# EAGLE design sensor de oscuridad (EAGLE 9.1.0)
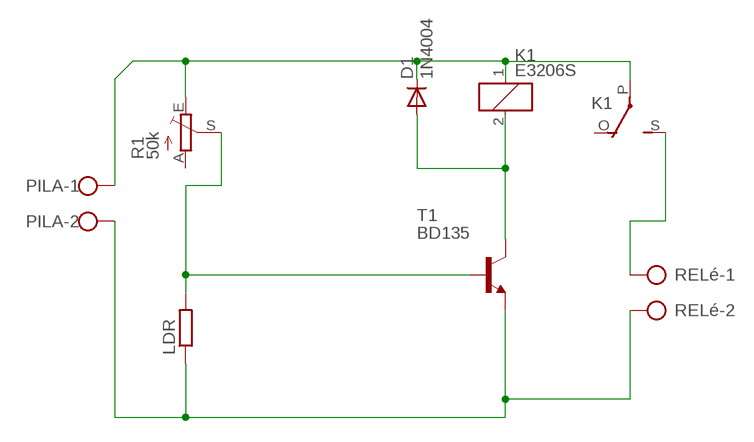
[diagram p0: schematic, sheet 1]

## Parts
D1  1N4004  [DO41-10]
K1  E3206S  [E3206S]
LDR  R-EU_0204/5  [0204/5]
PILA  AK500/2  [AK500/2]
R1  50k  TRIM_EU-CA9V  [CA9V]
RELé  AK500/2  [AK500/2]
T1  BD135  BD139  [TO126]

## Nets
GND: LDR.1 PILA.2 RELé.2 T1.1(E)
N$1: LDR.2 R1.S T1.3(B)
N$2: K1.S(2:S) RELé.1
N$4: D1.A K1.2 T1.2(C)
N$5: D1.K(C) K1.1 K1.P(2:P) PILA.1 R1.E
Unconnected: K1.O(2:O) R1.A

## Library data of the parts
D1 = diode:1N4004: DIODE
K1 = relay:E3206S: RELAY 1 x switch, Eichhoff/distributor Schukat
LDR = rcl:R-EU_: RESISTOR, European symbol
PILA = con-ptr500:AK500/2: CONNECTOR
R1 = pot:TRIM_EU-: POTENTIOMETER
RELé = con-ptr500:AK500/2: CONNECTOR; OC_FARNELL: unknown; OC_NEWARK: unknown
T1 = transistor-npn:BD139: NPN TRANSISTOR

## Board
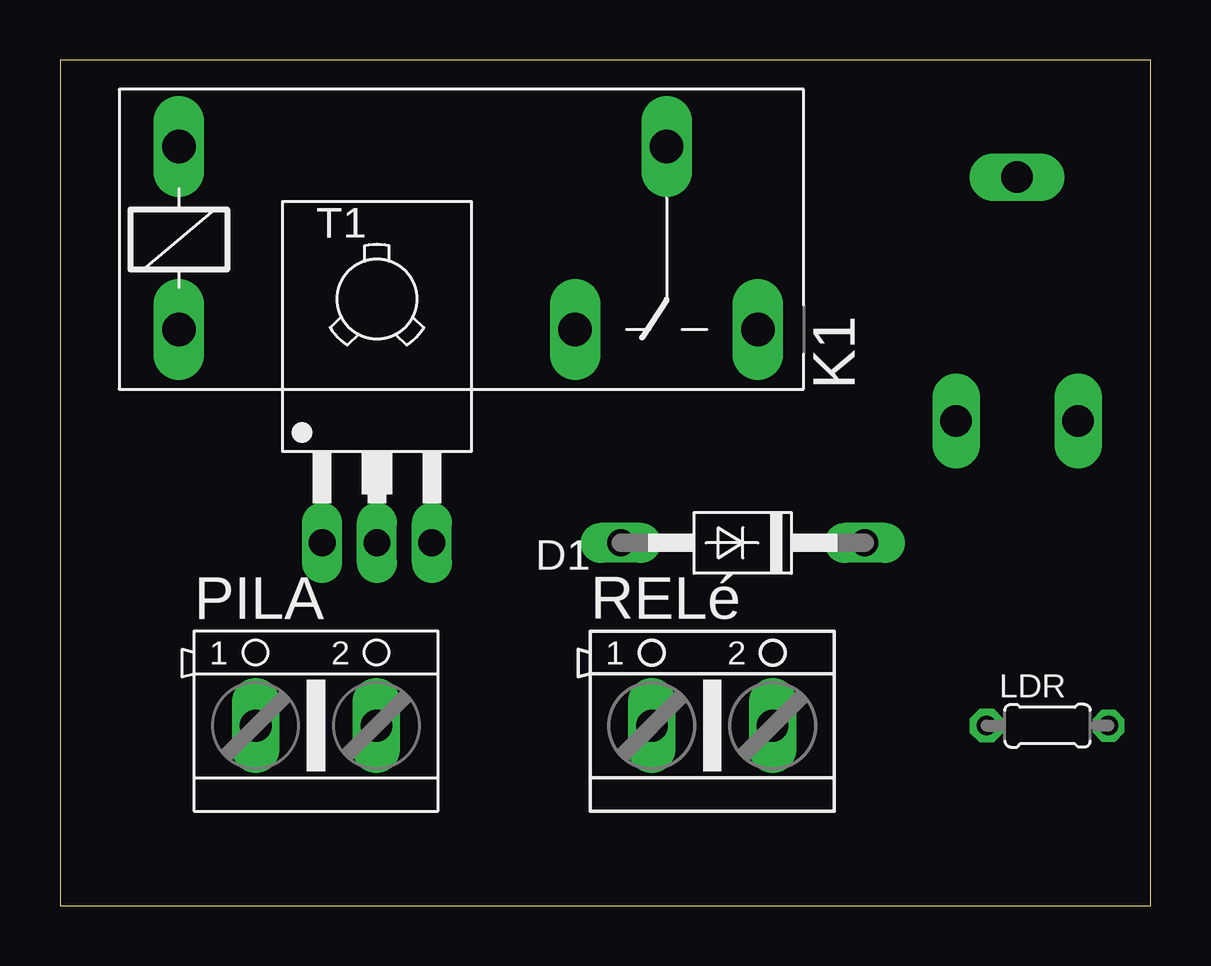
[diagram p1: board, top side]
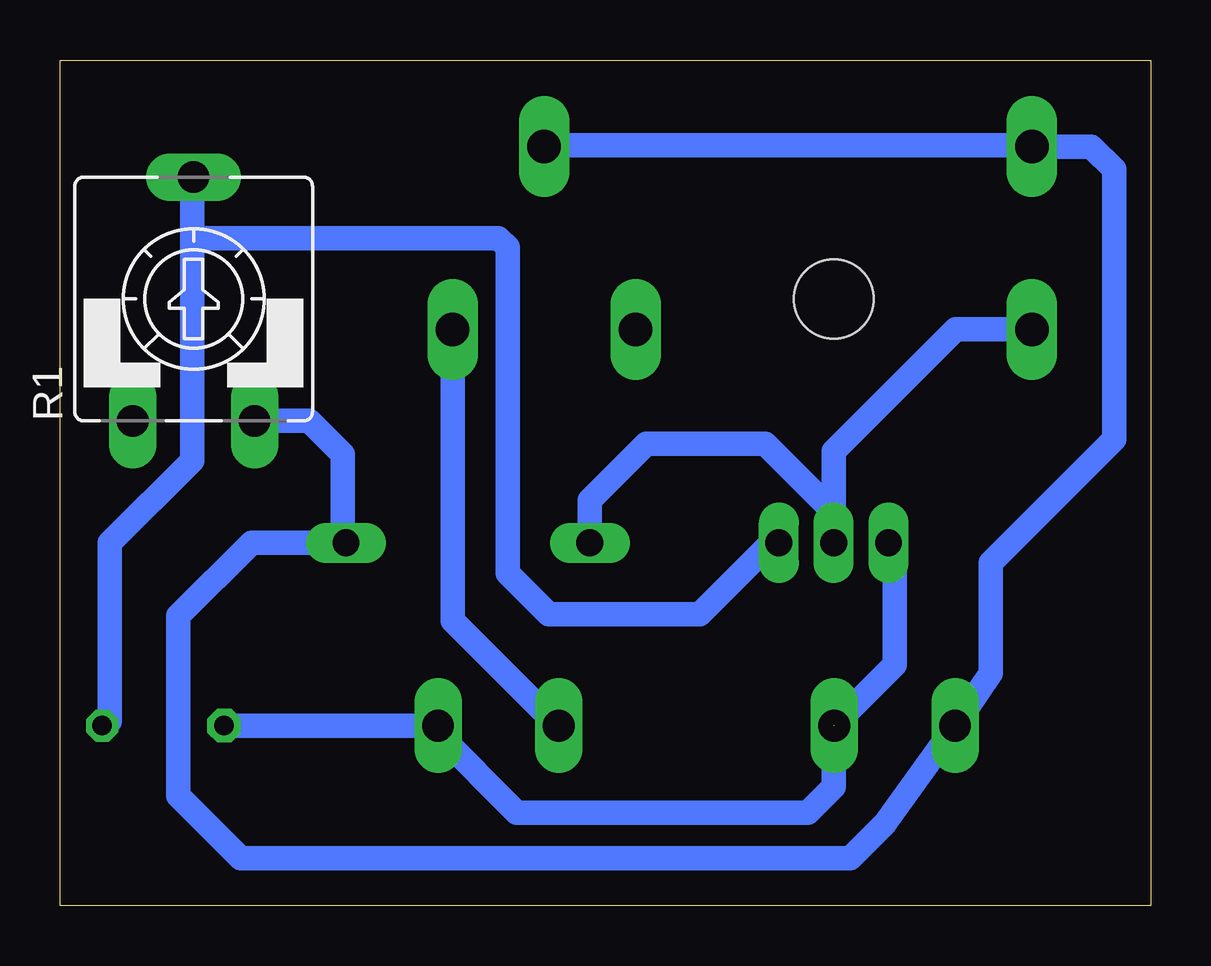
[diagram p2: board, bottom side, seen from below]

Size 45.45 x 35.23 mm. Coordinates in mm from the lower left corner, seen from the top.
Outline: 0,0 45.45,0 45.45,35.23 0,35.23 0,0
Copper layers (1*16): Top 0.035mm / dielectric 1.5mm / Bottom 0.035mm
Design rules "default *": minimum track width 25mil, minimum drill 0.35mm, track to track 20mil, track to pad 20mil, pad to pad 6mil, via to via 6mil, smd to smd 6mil, copper to edge 40mil, drill to drill 6mil, minimum pad ring 10mil, minimum via ring 8mil, stop-mask expansion 4mil, vias tented up to drill 0mil, thermal gap 10mil

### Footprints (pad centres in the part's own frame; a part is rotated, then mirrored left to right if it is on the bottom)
DO41-10 = drill 1.118 long: A 5.08,0; K -5.08,0
E3206S = drill 1.397 long: 1 -3.175,3.81; 2 -3.175,-3.81; O 13.335,-3.81; P 17.145,3.81; S 20.955,-3.81
0204/5 = drill 0.813 pad 1.397 octagon: 1 -2.54,0 | drill 0.813 octagon: 2 2.54,0
AK500/2 = drill 1.321 long: 1 -2.515,0; 2 2.515,0
CA9V = drill 1.321 long: A -2.54,-5.08; E 2.54,-5.08; S 0,5.08
TO126 = drill 1.118 long: 1 -2.286,-5.08; 2 0,-5.08; 3 2.286,-5.08 | hole 3.302: 0,5.08

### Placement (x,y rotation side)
D1  28.45,15.11 180 top
K1  8.13,27.81 0 top
LDR  41.15,7.49 0 top
PILA  10.67,7.49 0 top
R1  39.88,25.27 0 bottom
RELé  27.18,7.49 0 top
T1  13.21,20.19 0 top

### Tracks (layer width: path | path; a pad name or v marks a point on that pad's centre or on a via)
GND  (1 unrouted)
  Bottom 1.016: LDR.1 RELé.2 29.69,7.15 26.42,3.87 14.29,3.87 13.21,4.95 13.21,7.47 PILA.2 | T1.1 10.67,14.86 10.67,10.03 13.18,7.52
N$1
  Bottom 0.635: 43.37,7.68 LDR.2 | 39.94,29.97 R1.S
  Bottom 1.016: 43.37,7.68 43.37,15.11 39.94,18.54 39.94,27.81 | 39.94,29.97 39.94,27.81 | T1.3 15.81,15.11 18.8,12.13 25.08,12.13 26.8,13.84 26.8,27.43 27.18,27.81 39.94,27.81
N$2
  Bottom 0.635: 25.08,7.87 25.08,7.81
  Bottom 1.016: 25.08,7.87 29.08,11.88 K1.S | 25.08,7.81 RELé.1
N$4
  Bottom 0.635: 13.08,15.11 T1.2 13.08,16.26
  Bottom 1.016: D1.A 23.37,16.89 21.02,19.24 16.07,19.24 13.08,16.26 13.08,15.11 13.21,15.24 13.21,18.92 8.13,24 K1.2
N$5
  Bottom 0.635: 5.08,31.69 K1.1 | 33.66,15.11 D1.K
  Bottom 1.016: 5.08,31.69 25.08,31.69 K1.P | R1.E 35.05,20.19 33.66,18.8 33.66,15.11 37.47,15.11 40.51,12.06 40.51,4.57 37.91,1.97 12.51,1.97 11.07,3.4 PILA.1 6.67,9.68 6.67,14.29 1.52,19.43 1.52,30.67 2.48,31.62 K1.1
